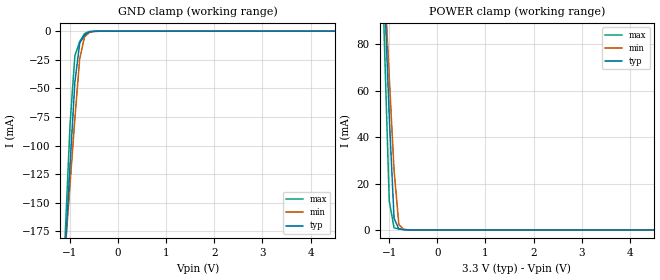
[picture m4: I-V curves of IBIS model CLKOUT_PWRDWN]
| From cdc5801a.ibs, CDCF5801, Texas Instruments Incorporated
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|   Clock Output  MODEL in POWER DOWN state
[Model]   CLKOUT_PWRDWN
Model_type   Terminator
|Signals   CLKOUT,CLKOUTB
|variable   typ   min   max
C_comp   2.9pF   NA   NA
[Temperature Range] 25.0   0   85.0
[Voltage range]   3.3V   3.135V   3.465V
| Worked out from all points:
|   GND clamp passes 1 mA (typ) near -0.61 V on its own axis
|   POWER clamp passes 1 mA (typ) near -0.81 V on its own axis
[GND Clamp]
|   40C:3.3V:nominal   85C:3.0V:weak   0C:3.6V:strong
|   Voltage   I(typ)   I(min)   I(max)
-3.6V     -2.068A    -1.638A    -2.609A
-1.1V     -191.3mA   -191.5mA   -177.1mA
-1V       -116.5mA   -133.7mA   -81.41mA
-900mV    -44.6mA    -76.39mA   -21.41mA
-800mV    -10.47mA   -24.23mA   -9.133mA
-700mV    -3.389mA   -4.973mA   -2.14mA
-600mV    -608.7uA   -1.147mA   -204.2uA
-500mV    -67.94uA   -176.9uA   -28.97uA
-300mV    -4.228uA   -4.461uA   -5.896uA
6.6V      90.78uA    69.83uA    129.7uA
[POWER Clamp]
|   40C:3.3V:nominal   85C:3.0V:weak   0C:3.6V:strong
|   Voltage   I(typ)   I(min)   I(max)
-3.6V     1.449A     1.143A     1.831A
-1.2V     156.3mA    148.7mA    150.2mA
-1.1V     102.5mA    107.3mA    80.16mA
-1V       48.84mA    65.9mA     12.51mA
-900mV    5.043mA    25.68mA    873.6uA
-800mV    395.6uA    2.294mA    462.2uA
-700mV    140.4uA    201.9uA    209.5uA
6.6V      -652.1pA   -3.956nA   -915pA
